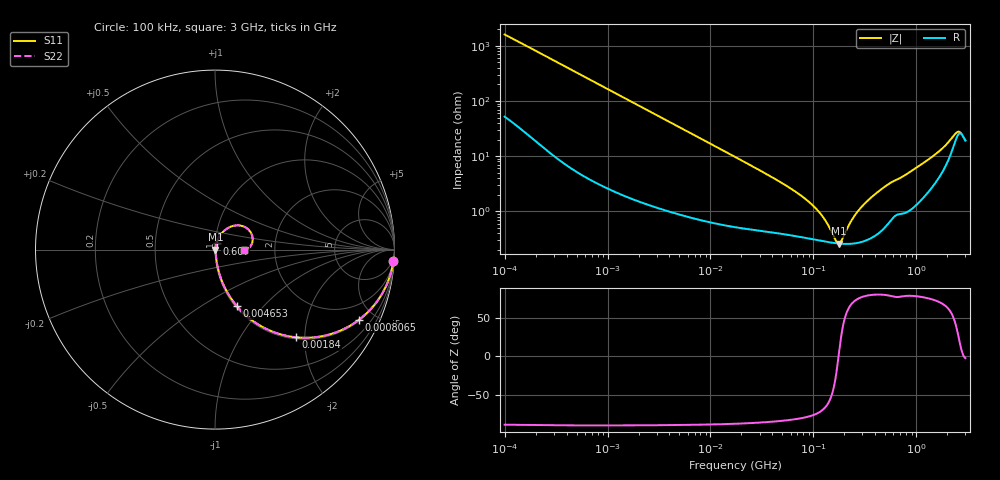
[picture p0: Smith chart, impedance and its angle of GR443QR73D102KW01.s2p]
!Murata Part Number: GR443QR73D102KW01
!These Parameters are Measured in Series Mode Connection
!Data Generated on Mar 13, 2026
!  o--ll--o
!Port1  Port2
!  o------o
!Operation Temp=25[degC], DC Bias Voltage=0[V]
!Freq. Start=100[kHz] Stop=3[GHz] 401[Steps]
# Hz S RI R 50
!Freq.(Hz) S11(Real) S11(Imag) S21(Real) S21(Imag) S12(Real) S12(Imag) S22(Real) S22(Imag)
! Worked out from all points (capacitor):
!   401 points, 100 kHz to 3 GHz, reference 50 ohm
!   read as one part in series: C = 983 pF near 105.3 kHz
!   lowest |Z| = 261 mohm at 176.2 MHz (marker M1)
!   series resonance near 175.6 MHz, so ESL is about 840 pH
!   S11 on the Smith chart (normalised r, x): 100 kHz: 2, -32; 806.5 kHz: 1.06, -4.08; 1.84 MHz: 1.03, -1.80; 4.653 MHz: 1.02, -0.72; 607 MHz: 1.02, +0.07; 3 GHz: 1.38, -0.01
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100000  0.9942 -0.0616  0.00583 0.0616  0.00583 0.0616  0.9942 -0.0616
246461  0.9749 -0.1465  0.0251 0.1465  0.0251 0.1465  0.9749 -0.1465
562235  0.8915 -0.3034  0.1085 0.3034  0.1085 0.3034  0.8915 -0.3034
806524  0.8029 -0.3902  0.1971 0.3902  0.1971 0.3902  0.8029 -0.3902
1839868  0.4486 -0.4886  0.5514 0.4886  0.5514 0.4886  0.4486 -0.4886
3161081  0.2219 -0.4049  0.7781 0.4049  0.7781 0.4049  0.2219 -0.4049
4652942  0.1202 -0.3128  0.8798 0.3128  0.8798 0.3128  0.1202 -0.3128
1.77727e7  0.0138 -0.0927  0.9862 0.0927  0.9862 0.0927  0.0138 -0.0927
5.523785e7  0.00455 -0.0282  0.9954 0.0282  0.9954 0.0282  0.00455 -0.0282
9.738194e7  0.00328 -0.0127  0.9967 0.0127  0.9967 0.0127  0.00328 -0.0127
1.260104e8  0.0029 -0.00696  0.9971 0.00696  0.9971 0.00696  0.0029 -0.00696
1.630551e8  0.00264 -0.00155  0.9974 0.00155  0.9974 0.00155  0.00264 -0.00155
1.761623e8  0.0026 6.67e-05  0.9974 -6.67e-05  0.9974 -6.67e-05  0.0026 6.67e-05
1.854806e8  0.00258 0.00115  0.9974 -0.00115  0.9974 -0.00115  0.00258 0.00115
2.339019e8  0.00261 0.00621  0.9974 -0.00621  0.9974 -0.00621  0.00261 0.00621
2.874592e8  0.00286 0.0111  0.9971 -0.0111  0.9971 -0.0111  0.00286 0.0111
5.475153e8  0.00725 0.0308  0.9928 -0.0308  0.9928 -0.0308  0.00725 0.0308
6.069703e8  0.00902 0.0341  0.991 -0.0341  0.991 -0.0341  0.00902 0.0341
1.616196e9  0.0472 0.1016  0.9528 -0.1016  0.9528 -0.1016  0.0472 0.1016
2.441062e9  0.1862 0.1119  0.8138 -0.1119  0.8138 -0.1119  0.1862 0.1119
2.637286e9  0.2104 0.0552  0.7896 -0.0552  0.7896 -0.0552  0.2104 0.0552
3e9  0.1612 -0.00497  0.8388 0.00497  0.8388 0.00497  0.1612 -0.00497
